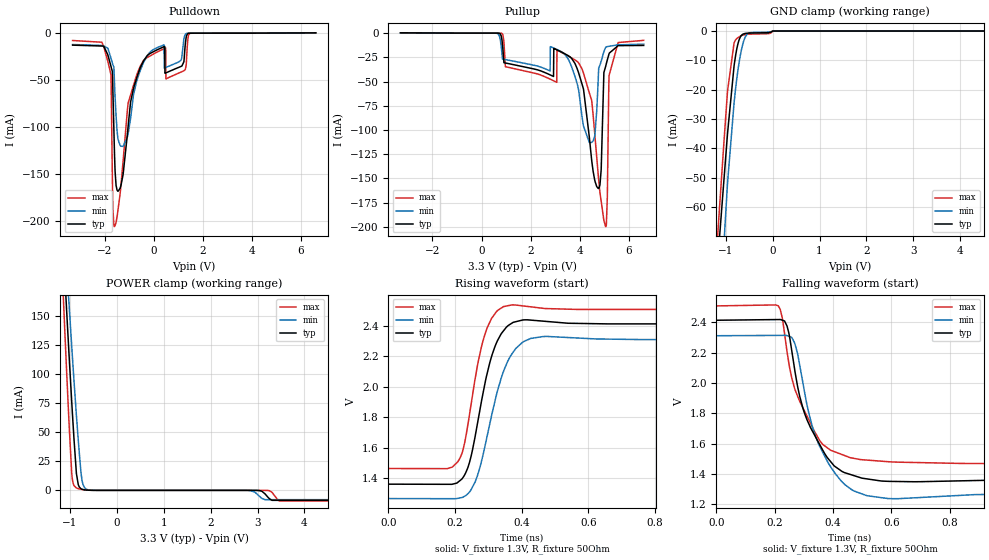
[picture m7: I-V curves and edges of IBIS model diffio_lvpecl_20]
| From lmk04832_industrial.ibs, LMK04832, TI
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|   diffio_lvpecl_20 Model
[Model]   diffio_lvpecl_20
Model_type   I/O
Polarity   Non-Inverting
Enable   Active-High
Vinl = 0.4
Vinh = 1.2
Vmeas = 1.8
Vref = 1.3
Cref = 1pF
Rref = 50
|   typ   min   max
C_comp   1.613pF   1.569pF   1.681pF
|  Where Nom  PVT is Nominal Process,   3.3V,  25C
|   Fast PVT is Strong Process,   3.45V, -40C
|   Slow PVT is Weak Process,   3.15V, 85C
[Model spec]
|subparameter
Vinl   0.400   0.370   0.430
Vinh   1.200   1.170   1.230
[Voltage Range]   3.3   3.15   3.45
|Junction Temperature
[Temperature Range]   25   85   -40
[Pullup Reference]   3.3   3.15   3.45
[Pulldown Reference]   0   0   0
[Power Clamp Reference]   3.3   3.15   3.45
[GND Clamp Reference]   0   0   0
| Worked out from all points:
|   GND clamp passes 1 mA (typ) near -0.62 V on its own axis
|   POWER clamp passes 1 mA (typ) near -0.74 V on its own axis
|   falling waveform, V_fixture 1.3V, R_fixture 50Ohm: 20-80 % time 101ps typ, 95.1ps min, 103ps max; typ from 2.41 V to 1.36 V
|   rising waveform, V_fixture 1.3V, R_fixture 50Ohm: 20-80 % time 59.3ps typ, 70.6ps min, 51.3ps max; typ from 1.36 V to 2.41 V
[Pulldown]
|   Voltage   I(typ)   I(min)   I(max)
-3.3V     -12.78mA   -12.13mA   -7.836mA
-2.11V    -13.7mA    -13.1mA    -9.669mA
-1.74V    -35.11mA   -26.46mA   -43.97mA
-1.66V    -61.59mA   -33.6mA    -186.5mA
-1.6V     -122.6mA   -49.83mA   -206mA
-1.49V    -167.2mA   -104mA     -195.6mA
-1.25V    -151.4mA   -120.6mA   -137.9mA
-1.04V    -99.29mA   -107.1mA   -74.51mA
-400mV    -29.07mA   -30.47mA   -28.65mA
500mV     -42.29mA   -36.48mA   -48.74mA
1.47V     -75.22uA   -51.23uA   -248.6uA
6.6V      325uA      298.6uA    356.9uA
[GND Clamp]
|   Voltage   I(typ)   I(min)   I(max)
-3.3V     -880.2mA   -824.9mA   -955.5mA
-1.18V    -80.5mA    -122.1mA   -71.85mA
-1.04V    -51.39mA   -73.25mA   -38.58mA
-960mV    -34.84mA   -51.71mA   -20.4mA
-820mV    -11.74mA   -24.32mA   -3.983mA
-730mV    -3.862mA   -12.43mA   -2.166mA
-670mV    -1.608mA   -6.896mA   -1.634mA
-620mV    -991.5uA   -3.63mA    -1.335mA
-570mV    -794.2uA   -1.677mA   -1.162mA
-500mV    -706.1uA   -676.8uA   -1.062mA
0V        0A         0A         0A
6.6V      0A         0A         0A
[Pullup]
|   Voltage   I(typ)   I(min)   I(max)
-3.3V     317.9uA    287.7uA    321.8uA
800mV     -2.925mA   -13.6mA    -86.17uA
970mV     -30.81mA   -27.28mA   -34.69mA
2.8V      -43.21mA   -13.91mA   -47.55mA
3.9V      -37.27mA   -52.89mA   -29.43mA
4.48V     -130.5mA   -112.8mA   -69.1mA
4.76V     -160.4mA   -40.82mA   -149.2mA
4.87V     -140.9mA   -29.02mA   -173.5mA
5.06V     -33.5mA    -14.53mA   -199.7mA
5.12V     -27.61mA   -13.9mA    -169.4mA
5.19V     -21.46mA   -13.59mA   -43.97mA
6.6V      -12.71mA   -11.4mA    -7.463mA
[POWER Clamp]
|   Voltage   I(typ)   I(min)   I(max)
-3.3V     1.944A     1.741A     2.257A
-1.23V    279.5mA    301.8mA    251.5mA
-1.11V    186.9mA    221.6mA    140.1mA
-1.07V    156.6mA    195.3mA    104.1mA
-1.01V    112.1mA    156.2mA    52.47mA
-960mV    76.51mA    124.5mA    14.98mA
-920mV    49.82mA    99.77mA    4.868mA
-860mV    14.5mA     64.71mA    2.062mA
-820mV    4.859mA    43.26mA    1.488mA
-740mV    963.9uA    8.663mA    758.6uA
-610mV    149uA      399.9uA    139uA
6.6V      -8.594mA   -8.021mA   -9.078mA
[Ramp]
R_load = 50
|   typ   min   max
dV/dt_r   0.629996/5.93093e-11   0.625399/7.05842e-11   0.62517/5.13114e-11
dV/dt_f   0.62998/1.00038e-10   0.625357/9.48237e-11   0.625469/1.0253e-10
[Falling Waveform]
V_fixture = 1.3V
V_fixture_min = 1.15V
V_fixture_max = 1.45V
R_fixture = 50Ohm
C_fixture = 0F
|   Time   V(typ)   V(min)   V(max)
0s        2.414V     2.312V     2.508V
212.6ps   2.418V     2.314V     2.509V
242.7ps   2.375V     2.312V     2.205V
258ps     2.222V     2.301V     2.041V
300.7ps   1.812V     1.961V     1.822V
335ps     1.664V     1.679V     1.688V
381.7ps   1.506V     1.48V      1.572V
464.5ps   1.394V     1.297V     1.506V
588ps     1.352V     1.239V     1.482V
10ns      1.364V     1.27V      1.466V
[Rising Waveform]
V_fixture = 1.3V
V_fixture_min = 1.15V
V_fixture_max = 1.45V
R_fixture = 50Ohm
C_fixture = 0F
|   Time   V(typ)   V(min)   V(max)
0s        1.363V     1.268V     1.465V
192ps     1.362V     1.268V     1.474V
220.6ps   1.397V     1.275V     1.563V
240.2ps   1.482V     1.303V     1.773V
270.3ps   1.795V     1.44V      2.172V
297.8ps   2.099V     1.691V     2.392V
319.4ps   2.26V      1.901V     2.477V
347.8ps   2.372V     2.113V     2.526V
404.1ps   2.437V     2.293V     2.529V
10ns      2.413V     2.311V     2.507V
